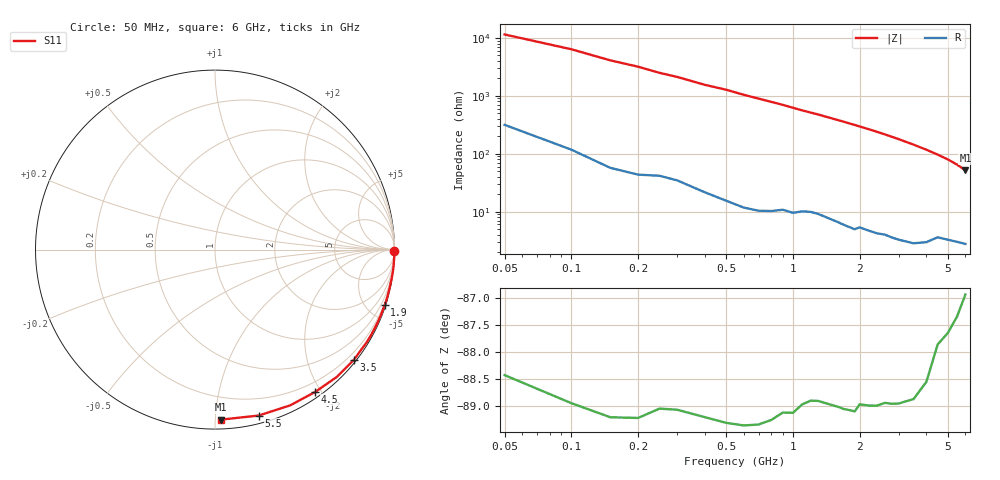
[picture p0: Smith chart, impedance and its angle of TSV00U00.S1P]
! SIEMENS Small Signal Semiconductors
! BAT14-03W
! Si Schottky Diode in SOD323
! VR = 0 V
! S-Parameters:  November  1995
# GHz  S  MA  R  50
!  f  S11
! GHz  MAG  ANG
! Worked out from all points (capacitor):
!   34 points, 50 MHz to 6 GHz, reference 50 ohm
!   read as one part to ground: C = 259 fF near 50 MHz
!   lowest |Z| = 51.8 ohm at 6 GHz (marker M1)
!   S11 on the Smith chart (normalised r, x): 50 MHz: open; 1.9 GHz: 0.10, -6.28; 3.5 GHz: 0.06, -2.87; 4.5 GHz: 0.07, -1.93; 5.5 GHz: 0.06, -1.30; 6 GHz: 0.06, -1.03
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0.05  0.9998 -0.5
0.1  0.9997 -0.9
0.15  0.9997 -1.4
0.2  0.9996 -1.8
0.25  0.9993 -2.3
0.3  0.9992 -2.7
0.4  0.9991 -3.7
0.5  0.999 -4.5
0.6  0.9989 -5.5
0.8  0.9983 -7.3
0.9  0.9978 -8.2
1.1  0.9968 -10.2
1.3  0.996 -12.0
1.6  0.9955 -15.0
1.7  0.9954 -16.0
1.8  0.9952 -17.1
1.9  0.9951 -18.1
2.2  0.9936 -21.4
2.4  0.9929 -23.7
2.6  0.9919 -26.1
2.8  0.9913 -28.7
3  0.9905 -31.3
3.5  0.9878 -38.4
4  0.9819 -46.2
4.5  0.9699 -54.8
5  0.9637 -64.2
5.5  0.9562 -75.2
6  0.9479 -88.0
